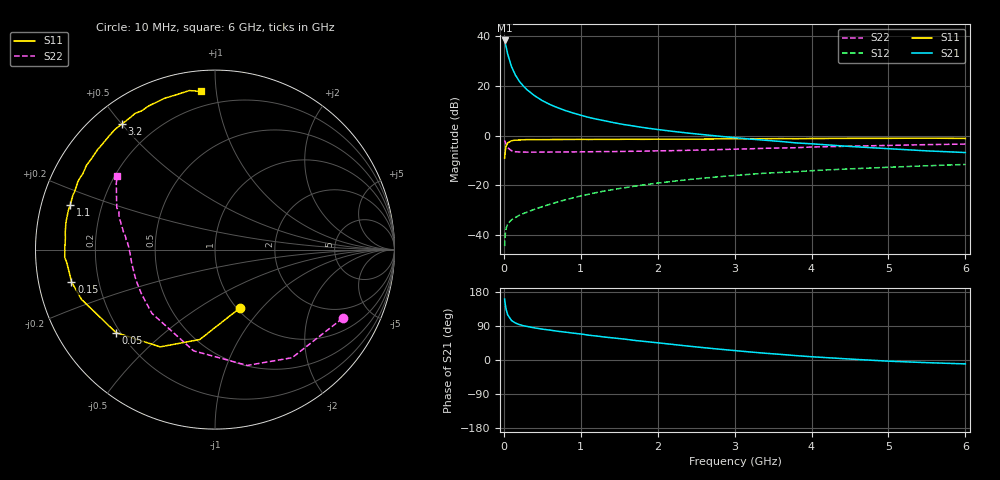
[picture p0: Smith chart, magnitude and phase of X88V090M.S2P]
! SIEMENS Small Signal Semiconductors
! BFP136W
! Si NPN RF Bipolar Junction Transistor in SOT343
! VCE = 8 V  IC = 90 mA
! Common Emitter S-Parameters:  September  1994
# GHz  S  MA  R  50
!  f  S11  S21  S12  S22
! GHz  MAG  ANG  MAG  ANG  MAG  ANG  MAG  ANG
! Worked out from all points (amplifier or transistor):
!   40 points, 10 MHz to 6 GHz, reference 50 ohm
!   highest |S21| = 38.4 dB at 10 MHz (marker M1)
!   |S21| within 3 dB of that: start of sweep to 32.42 MHz
!   unconditionally stable (mu >= 1): 622.4 MHz to 2.973 GHz
!   at 200 MHz: K = 0.62, MSG = 27.0 dB, |S12| = -32.0 dB
!   at 1.5 GHz: K = 1.10, MAG = 11.1 dB, |S12| = -21.2 dB
!   at 6 GHz: K = 0.95, MSG = 2.4 dB, |S12| = -11.5 dB
!   S11 on the Smith chart (normalised r, x): 10 MHz: 1.03, -0.77; 50 MHz: 0.18, -0.35; 150 MHz: 0.10, -0.11; 1.1 GHz: 0.09, +0.15; 3.2 GHz: 0.09, +0.50; 6 GHz: 0.11, +0.91
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0.01  0.3538 -66.9  83.04 160.9  0.006 70.1  0.8073 -28.3
0.02  0.5081 -99.6  71.76 144.9  0.0107 57.9  0.7398 -54.5
0.03  0.622 -119.4  61.16 133.4  0.0137 49.6  0.6699 -74.4
0.05  0.7198 -140.0  44.09 119.1  0.0168 39.3  0.5767 -101.9
0.1  0.7941 -159.6  24.59 104.2  0.0204 34.6  0.4997 -134.7
0.15  0.8196 -167.4  16.75 97.6  0.0226 37.1  0.4785 -148.5
0.2  0.8224 -171.6  12.6 93.6  0.0251 38.4  0.4726 -156.2
0.25  0.8293 -175.0  10.17 90.7  0.0271 41.1  0.4706 -161.0
0.3  0.8384 -177.1  8.504 88.6  0.0289 42.9  0.469 -164.3
0.4  0.8362 178.6  6.409 84.7  0.0332 47.3  0.4692 -168.7
0.5  0.836 175.6  5.11 81.4  0.0375 49.7  0.4702 -171.7
0.6  0.8398 173.4  4.266 78.9  0.0418 52.2  0.471 -173.7
0.7  0.8427 170.7  3.677 75.9  0.0467 54.2  0.4724 -175.1
0.8  0.8444 168.9  3.219 73.5  0.0514 55.5  0.473 -176.5
0.9  0.8442 167.2  2.877 70.9  0.0563 56.3  0.474 -177.8
1.1  0.8438 162.7  2.352 65.5  0.0664 57.4  0.477 -179.5
1.5  0.8481 155.9  1.75 56.6  0.0868 57.3  0.4833 177.4
2.2  0.8548 143.5  1.227 41.0  0.1214 53.4  0.5022 172.2
3.2  0.8713 126.5  0.859 21.2  0.1677 44.8  0.5474 163.7
4.5  0.8888 108.4  0.61 2.5  0.216 33.7  0.6178 152.6
5.5  0.8978 99.2  0.497 -7.0  0.2492 25.6  0.6641 145.9
6  0.8842 94.9  0.46 -10.3  0.2652 21.3  0.6809 143.0
